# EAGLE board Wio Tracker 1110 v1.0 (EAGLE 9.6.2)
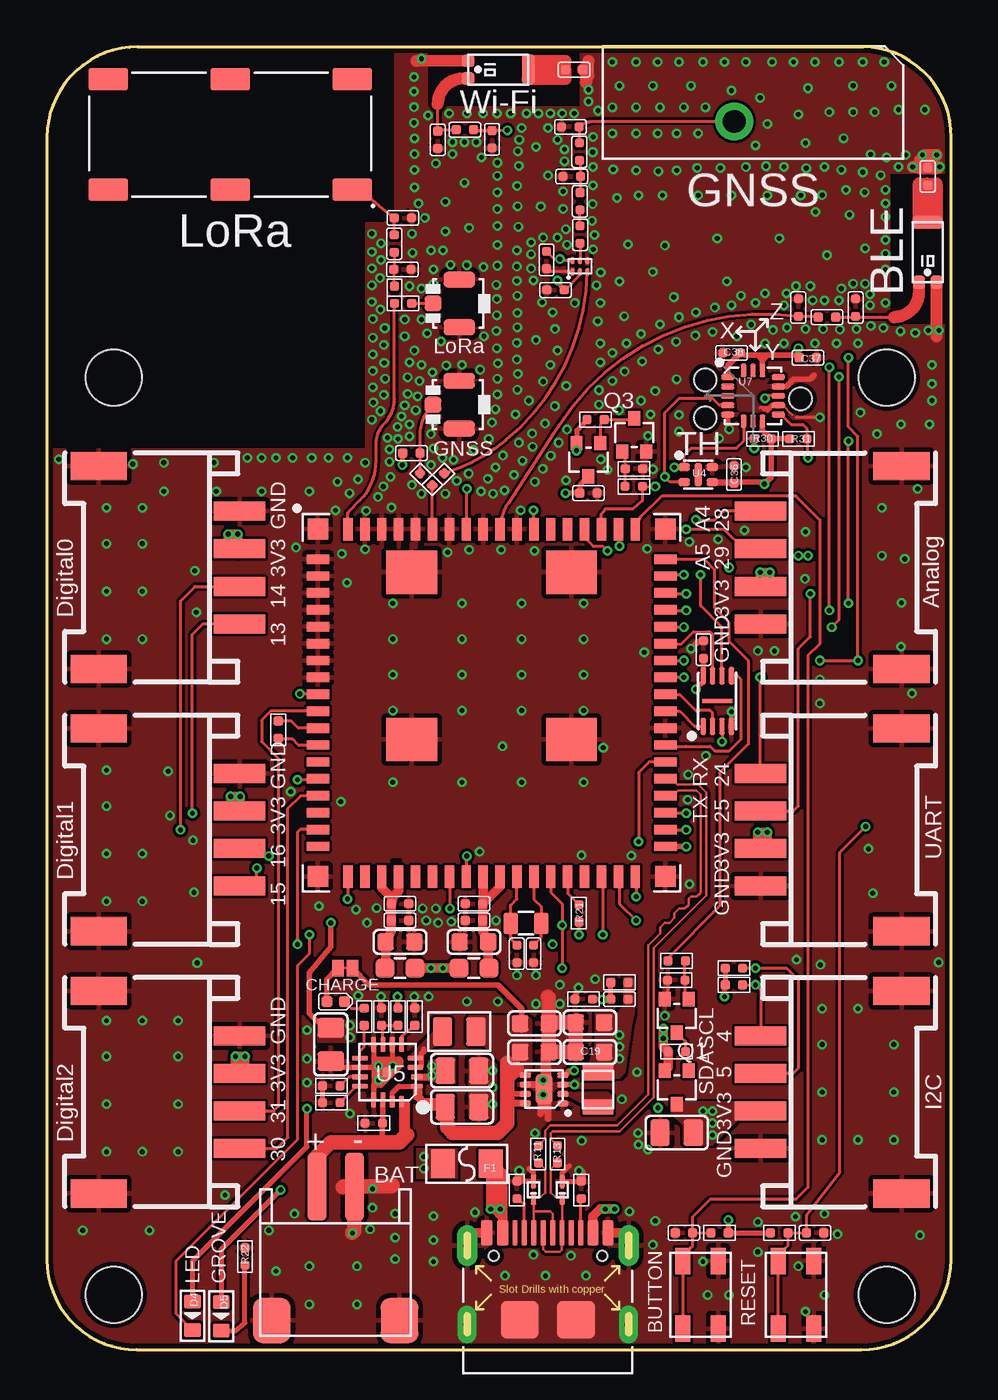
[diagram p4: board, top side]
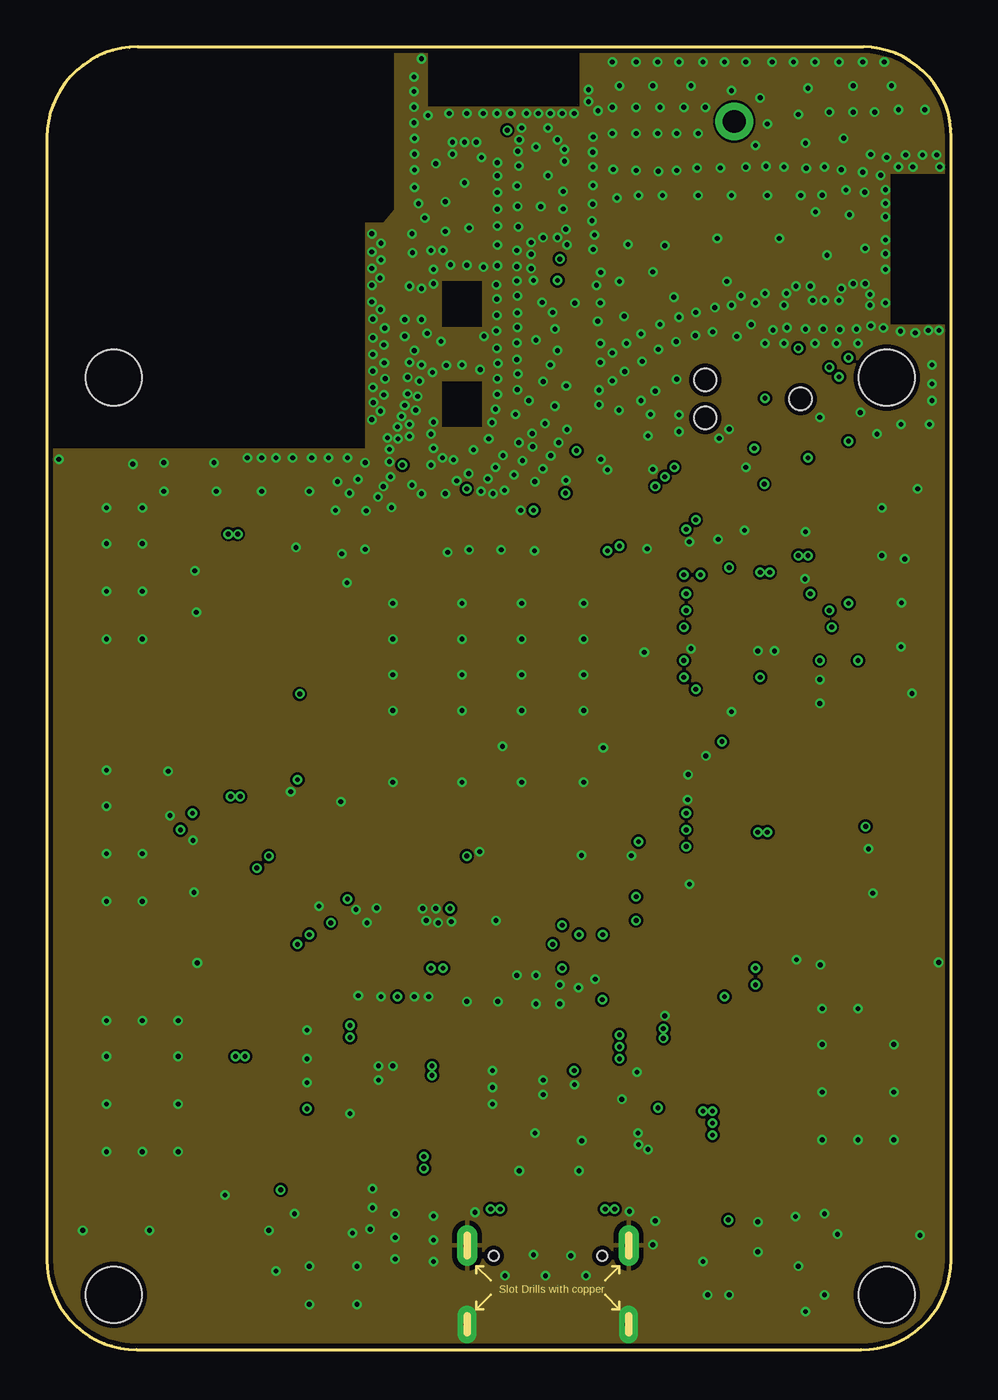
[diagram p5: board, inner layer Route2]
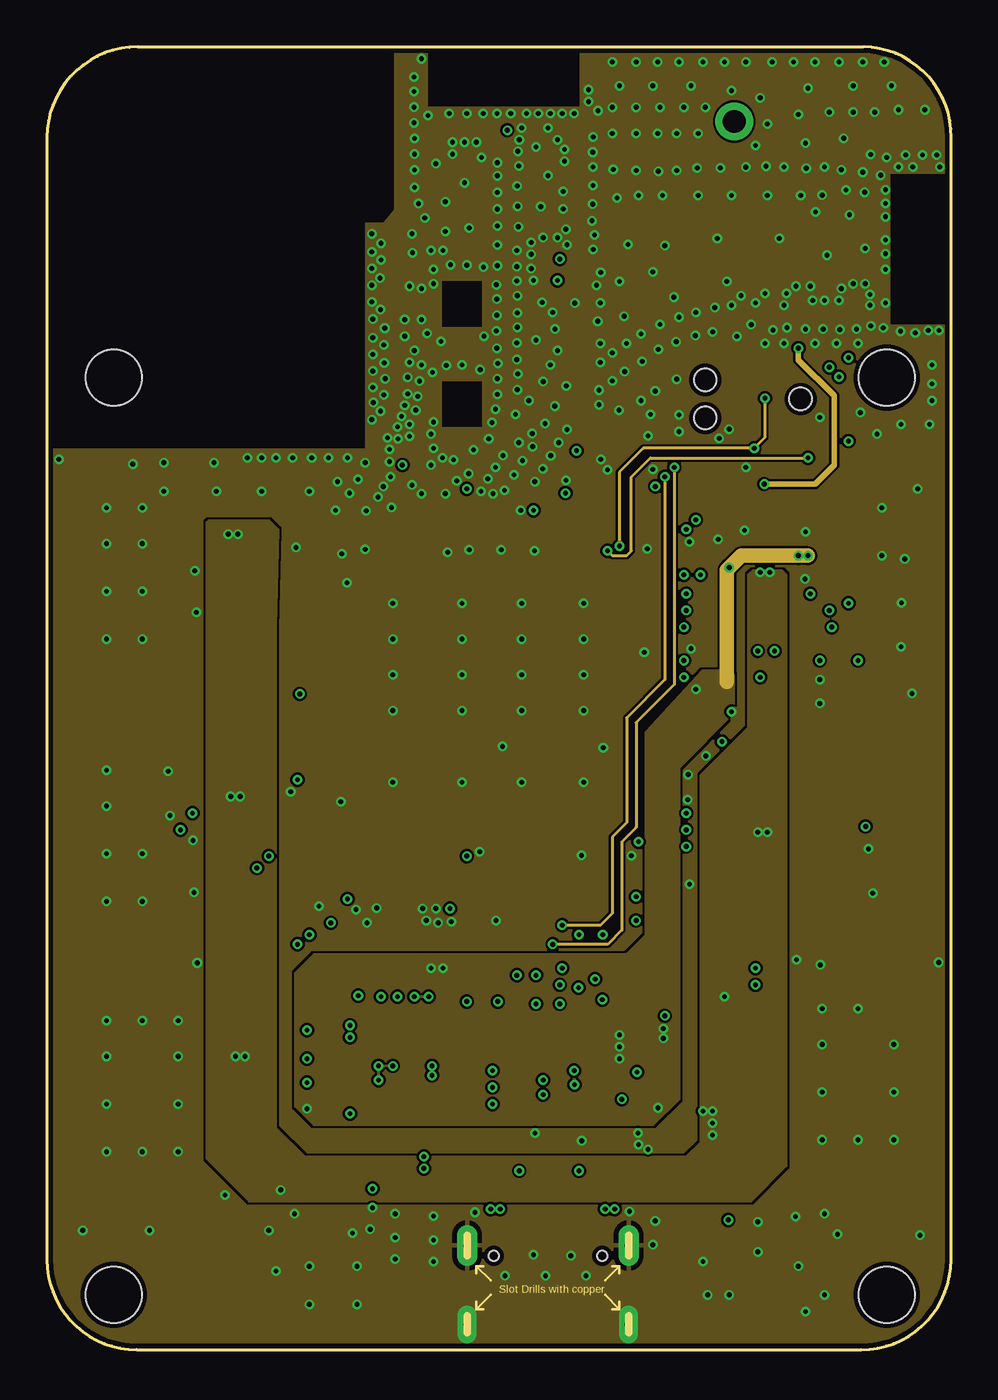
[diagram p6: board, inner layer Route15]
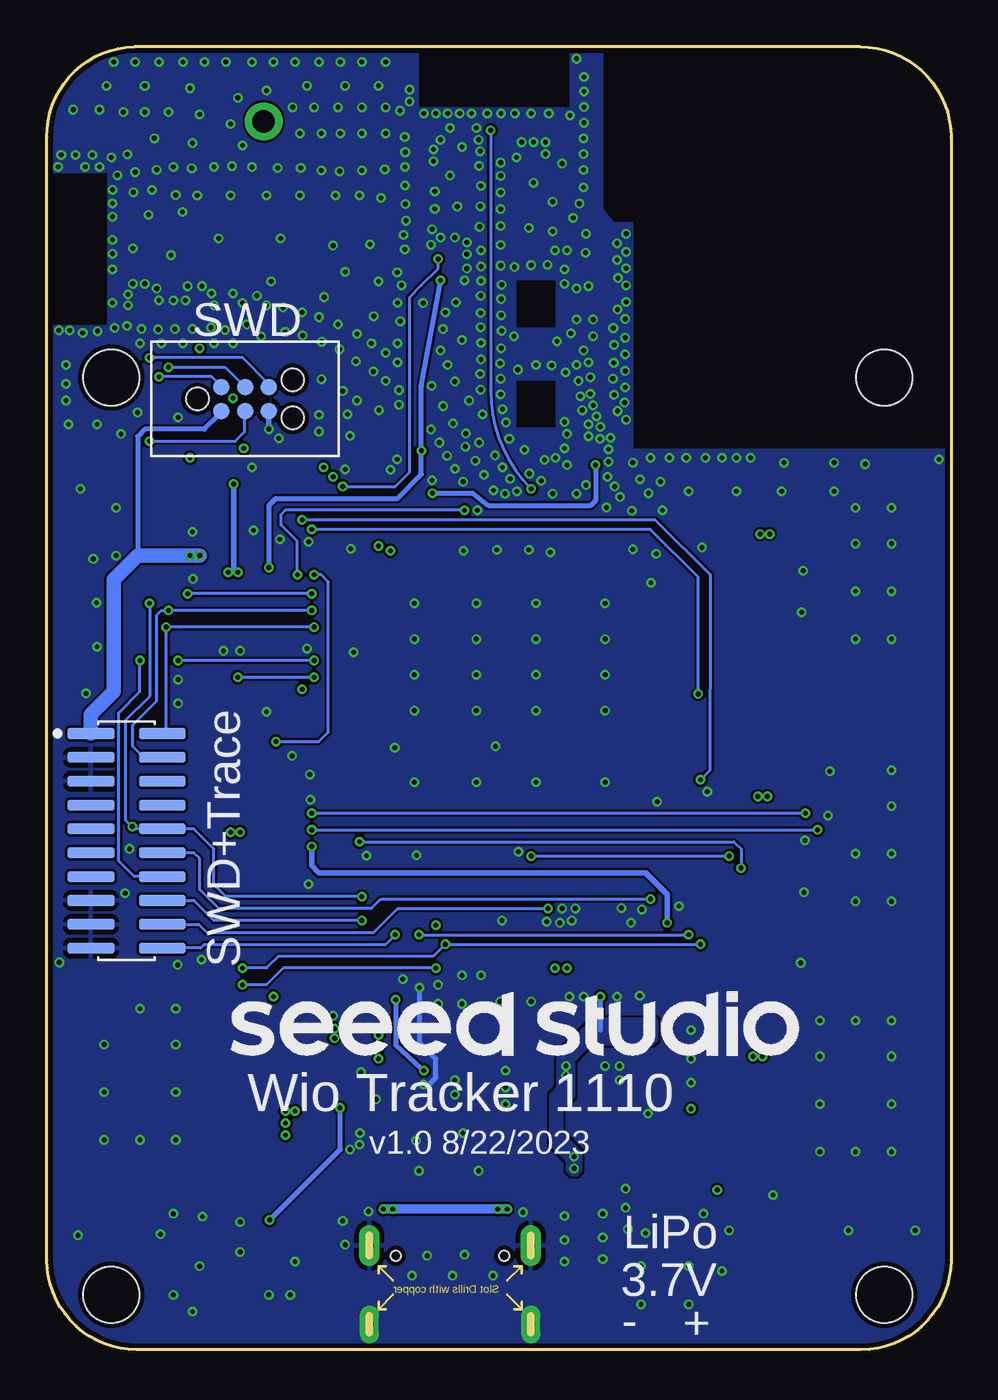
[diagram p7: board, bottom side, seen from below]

Size 48.13 x 69.38 mm. Coordinates in mm from the lower left corner, seen from the top.
Outline: 0,64.58 0,4.78 arc90 4.78,0 43.35,0 arc90 48.13,4.78 48.13,64.58 arc90 43.48,69.38 4.83,69.38 arc90 0,64.58
Copper layers (1*2*15*16): Top 0.035mm / dielectric 0.2mm / Route2 0.0175mm / dielectric 0.3mm / Route15 0.0175mm / dielectric 0.2mm / Bottom 0.035mm
Design rules "SeeedStudio_4layer_DRU_no_angle_20140221 *": minimum track width 1mil, minimum drill 10mil, track to track 5mil, track to pad 5mil, pad to pad 5mil, via to via 5mil, smd to smd 0mil, copper to edge 10mil, drill to drill 8mil, minimum pad ring 4mil, minimum via ring 4mil, stop-mask expansion 4mil, vias tented up to drill 25mil, thermal gap 10mil
Holes 3 mm at 3.56,2.92 44.7,2.92 3.56,51.77 44.7,51.77
tRestrict: area 18.4,24.5 to 18.8,26

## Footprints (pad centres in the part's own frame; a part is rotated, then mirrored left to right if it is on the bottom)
U-FL3P-SMD-2.6X2.6X1.0MM = smd 0.889 x 0.838: D -1.397,0 | smd 1.676 x 0.838: GND1 0,1.27; GND2 0,-1.27
ANT-SMD3P-3.1X1.6X1.04MM = smd 0.65 x 0.7: 1 -0.47,1.6; 2 0.47,1.6 | smd 1.6 x 0.7: 3 0,-1.6
ANT-DIP-14X6X4MM = drill 1.2 pad 2: 1 -1,-1
ANT6-SMD-15X6.5X1.63MM = smd 2.1 x 1.2: 1 -6.5,2.95; 2 0,2.95; 3 6.5,2.95; 4 6.5,-2.95; 5 0,-2.95; 6 -6.5,-2.95
C0402 = smd 0.5 x 0.5: 1 -0.463,0; 2 0.463,0
C0603 = smd 0.889 x 0.889: 1 -0.762,0; 2 0.762,0
C0805 = smd 1.016 x 1.397: 1 -0.889,0; 2 0.889,0
R0402 = smd 0.5 x 0.5: 1 -0.463,0; 2 0.463,0
H2X10-1.27-12.7X3X5.7MM = smd 0.6 x 2.5: 1 -5.715,-1.9; 2 -5.715,1.9; 3 -4.445,-1.9; 4 -4.445,1.9; 5 -3.175,-1.9; 6 -3.175,1.9; 7 -1.905,-1.9; 8 -1.905,1.9; 9 -0.635,-1.9; 10 -0.635,1.9; 11 0.635,-1.9; 12 0.635,1.9; 13 1.905,-1.9; 14 1.905,1.9; 15 3.175,-1.9; 16 3.175,1.9; 17 4.445,-1.9; 18 4.445,1.9; 19 5.715,-1.9; 20 5.715,1.9
SOD-923 = smd 0.7 x 0.3: 1 -0.45,0; 2 0.45,0
LED-0402 = smd 0.58 x 0.58: + -0.468,0; - 0.468,0
LED-0603 = smd 0.762 x 0.889: + -0.762,0; - 0.762,0
FS1206 = smd 1.27 x 1.524: 1 -1.27,0; 2 1.27,0
F0603 = smd 1 x 1: 1 -0.8,0; 2 0.8,0
CONNECTER6P-1.27-9.9X6.1MM = smd 0.88 x 0.88: 1 -1.27,-0.635; 2 -1.27,0.635; 3 0,-0.635; 4 0,0.635; 5 1.27,-0.635; 6 1.27,0.635 | hole 1.2: -2.54,0; 2.54,1.016; 2.54,-1.016
HW2-SMD-2.0-90D = smd 2 x 2.4: 3 3.4,-2.181; 4 -3.4,-2.181 | smd 1 x 3.6: + -1,4.953; - 1,4.953
HW4-SMD-2.0-90D = smd 1.01 x 2.74: 1 -3,-0.1; 2 -1,-0.1; 3 1,-0.1; 4 3,-0.1 | smd 1.5 x 3: SS1 -5.4,7.4; SS2 5.4,7.4
2P-SMD-SHORT = smd 0.61 x 0.889: 1 -0.381,0; 2 0.381,0
SW4P-SMD-4.5X3.2X2.5MM = smd 1.4 x 0.8: 1 -1.8,-0.94; 2 1.8,-0.94; 3 1.8,0.94; 4 -1.8,0.94
L0402 = smd 0.5 x 0.5: 1 -0.463,0; 2 0.463,0
L0806 = smd 1.016 x 1.524: 1 -0.889,0; 2 0.889,0
L201610@1 = smd 0.8 x 1.6: 1 -0.9,0; 2 0.9,0
SOT-323 = smd 0.762 x 0.635: 1 0.889,-0.635; 2 0.889,0.635; 3 -0.889,0
MODULE72_0D9_20X20X2MM = smd 1.2 x 0.5: 1 -9.25,7.65; 2 -9.25,6.75; 3 -9.25,5.85; 4 -9.25,4.95; 5 -9.25,4.05; 6 -9.25,3.15; 7 -9.25,2.25; 8 -9.25,1.35; 9 -9.25,0.45; 10 -9.25,-0.45; 11 -9.25,-1.35; 12 -9.25,-2.25; 13 -9.25,-3.15; 14 -9.25,-4.05; 15 -9.25,-4.95; 16 -9.25,-5.85; 17 -9.25,-6.75; 18 -9.25,-7.65; 37 9.25,-7.65; 38 9.25,-6.75; 39 9.25,-5.85; 40 9.25,-4.95; 41 9.25,-4.05; 42 9.25,-3.15; 43 9.25,-2.25; 44 9.25,-1.35; 45 9.25,-0.45; 46 9.25,0.45; 47 9.25,1.35; 48 9.25,2.25; 49 9.25,3.15; 50 9.25,4.05; 51 9.25,4.95; 52 9.25,5.85; 53 9.25,6.75; 54 9.25,7.65 | smd 0.5 x 1.2: 19 -7.65,-9.25; 20 -6.75,-9.25; 21 -5.85,-9.25; 22 -4.95,-9.25; 23 -4.05,-9.25; 24 -3.15,-9.25; 25 -2.25,-9.25; 26 -1.35,-9.25; 27 -0.45,-9.25; 28 0.45,-9.25; 29 1.35,-9.25; 30 2.25,-9.25; 31 3.15,-9.25; 32 4.05,-9.25; 33 4.95,-9.25; 34 5.85,-9.25; 35 6.75,-9.25; 36 7.65,-9.25; 55 7.65,9.25; 56 6.75,9.25; 57 5.85,9.25; 58 4.95,9.25; 59 4.05,9.25; 60 3.15,9.25; 61 2.25,9.25; 62 1.35,9.25; 63 0.45,9.25; 64 -0.45,9.25; 65 -1.35,9.25; 66 -2.25,9.25; 67 -3.15,9.25; 68 -4.05,9.25; 69 -4.95,9.25; 70 -5.85,9.25; 71 -6.75,9.25; 72 -7.65,9.25 | smd 1.1 x 1.1: 73 -9.25,9.25; 74 -9.25,-9.25; 75 9.25,-9.25; 76 9.25,9.25 | smd 2.7 x 2.3: 77 -4.25,6.95; 78 -4.25,-1.95; 79 4.25,-1.95; 80 4.25,6.95
USON8-0.5-3X2MM = smd 0.9 x 0.3: 1 -1.35,0.75; 2 -1.35,0.25; 3 -1.35,-0.25; 4 -1.35,-0.75; 5 1.35,-0.75; 6 1.35,-0.25; 7 1.35,0.25; 8 1.35,0.75 | smd 0.2 x 1.6: BP 0,0
BGA6-0.4-1.1X0.7X0.4MM = smd 0.4 x 0.2: 1 -0.3,0.4; 2 -0.3,0; 3 -0.3,-0.4; 4 0.3,-0.4; 5 0.3,0; 6 0.3,0.4
SNR4-0.8-1.5X1.5X0.54MM = smd 0.6 x 0.4: 1 -0.75,0.4; 2 -0.75,-0.4; 3 0.75,-0.4; 4 0.75,0.4 | smd 0.4 x 1.2: 5 0,0
QFN16G-0.5-3X3MM = smd 0.65 x 0.28: 1 -1.575,0.75; 2 -1.575,0.25 | smd 0.85 x 0.28: 3 -1.475,-0.25; 4 -1.475,-0.75; 9 1.475,-0.75; 10 1.475,-0.25; 11 1.475,0.25; 12 1.475,0.75 | smd 0.28 x 0.85: 5 -0.75,-1.475; 6 -0.25,-1.475; 7 0.25,-1.475; 8 0.75,-1.475; 13 0.75,1.475; 14 0.25,1.475 | smd 0.28 x 0.65: 15 -0.25,1.575; 16 -0.75,1.575 | smd 0.508 x 0.508: PAD 0,0
DFN8G-0.5-2X2MM = smd 0.6 x 0.3: 1 -1,0.75; 2 -1,0.25; 3 -1,-0.25; 4 -1,-0.75; 5 1,-0.75; 6 1,-0.25; 7 1,0.25; 8 1,0.75 | smd 0.9 x 1.6: 9 0,0
LGA16-0.5-3X3MM = smd 0.7 x 0.3: 1 -1.35,0.873; 2 -1.35,0.373; 3 -1.35,-0.127; 4 -1.35,-0.627; 5 -1.35,-1.127; 9 1.35,-1.127; 10 1.35,-0.627; 11 1.35,-0.127; 12 1.35,0.373; 13 1.35,0.873 | smd 0.3 x 0.7: 6 -0.5,-1.477; 7 0,-1.477; 8 0.5,-1.477; 14 0.5,1.223; 15 0,1.223; 16 -0.5,1.223
USB2.0-TYPE-C = smd 1.35 x 0.6: A1_B12 0.125,3.25; A4_B9 0.125,2.4; B1_A12 0.125,-3.2; B4_A9 0.125,-2.4 | smd 1.35 x 0.3: A5 0.125,1.25; A6 0.125,0.25; A7 0.125,-0.25; A8 0.125,-1.25; B5 0.125,-1.75; B6 0.125,-0.75; B7 0.125,0.75; B8 0.125,1.75 | drill 0.4 pad 1 long: S1 -4.75,4.3; S2 -4.75,-4.3 | drill 0.4 pad 1.1 long: S3 -0.55,4.3; S4 -0.55,-4.3 | smd 2 x 2: S5 -4.5,1.5; S6 -4.5,-1.5 | hole 0.55: -1.1,-2.89; -1.1,2.89
X2-SMD-L2.0X1.2X0.55MM = smd 0.762 x 1.143: 1 -0.813,0; 2 0.813,0

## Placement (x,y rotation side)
ANT1  U.FL-R-SMT-1  [U-FL3P-SMD-2.6X2.6X1.0MM]  21.95,55.72 0 top
ANT2  U.FL-R-SMT-1  [U-FL3P-SMD-2.6X2.6X1.0MM]  21.94,50.33 0 top
ANT3  RFECA3216060A1T  [ANT-SMD3P-3.1X1.6X1.04MM]  24.03,68.17 90 top
ANT4  RFECA3216060A1T  [ANT-SMD3P-3.1X1.6X1.04MM]  46.89,58.45 180 top
ANT5  M04-0103010R0A  [ANT-DIP-14X6X4MM]  37.59,66.42 0 top
ANT6  MD1506  [ANT6-SMD-15X6.5X1.63MM]  9.75,64.72 180 top
C1  7.5pF  [C0402]  18.92,57.53 180 top
C2  DNP  [C0402]  18.95,60.27 180 top
C3  1.2pF  [C0402]  27.94,62.48 0 top
C4  DNP  [C0402]  27.86,65.12 0 top
C5  1.2pF  [C0402]  23.7,64.46 90 top
C6  0.5pF  [C0402]  20.8,64.44 90 top
C7  1.2pF  [C0402]  40.01,55.5 270 top
C8  0.5pF  [C0402]  43.05,55.5 270 top
C9  1nF  [C0402]  28.07,68.17 180 top
C10  1nF  [C0402]  46.89,62.48 270 top
C11  47pF  [C0402]  22.73,23.75 0 top
C12  100nF  [C0402]  22.73,22.86 0 top
C13  10uF  [C0603]  22.73,21.72 0 top
C14  47pF  [C0402]  18.8,22.86 180 top
C15  100nF  [C0402]  18.8,23.75 180 top
C16  10uF  [C0603]  18.8,21.72 180 top
C17  12pF  [C0402]  25.02,21.08 90 top
C18  10uF  [C0805]  33.53,11.56 180 top
C19  10uF  [C0603]  28.91,15.85 0 top
C20  12pF  [C0402]  25.91,21.08 90 top
C21  10uF  [C0603]  25.96,17.37 180 top
C22  10uF  [C0805]  22.1,14.86 0 top
C23  10uF  [C0805]  15.11,16.26 270 top
C24  10uF  [C0805]  22.1,12.93 0 top
C25  1uF  [R0402]  17.4,12.06 180 top
C26  10uF  [C0603]  28.91,17.42 0 top
C27  10uF  [C0603]  25.96,15.85 180 top
C28  100nF  [C0402]  33.91,6.22 0 top
C29  100nF  [C0402]  40.89,6.22 180 top
C30  100nF  [C0402]  34.95,37.29 270 top
C31  1nF  [C0402]  27.08,56.44 0 top
C32  1nF  [C0402]  26.59,58.04 90 top
C33  100nF  [C0402]  28.83,45.62 180 top
C34  1nF  [C0402]  28.37,61.16 270 top
C35  1nF  [C0402]  30.48,18.67 0 top
C36  100nF  [C0402]  36.58,46.61 270 top
C37  100nF  [C0402]  40.51,52.83 180 top
C38  100nF  [C0402]  36.45,53.09 0 top
CN1  DNP  [H2X10-1.27-12.7X3X5.7MM]  43.89,27.1 270 bottom
D1  DF2S6.8FS  [SOD-923]  27.43,8.51 90 top
D2  DF2S6.8FS  [SOD-923]  25.91,8.51 90 top
D3  Green  [LED-0402]  15.37,18.54 0 top
D4  Blue  [LED-0603]  7.75,1.8 270 top
D5  Red  [LED-0603]  9.27,1.78 270 top
F1  750mA  [FS1206]  22.35,9.91 180 top
FB1  BLM18PG121SN1D  [F0603]  22.73,20.32 180 top
FB2  BLM18PG121SN1D  [F0603]  18.8,20.32 0 top
FR1  SEEEDSTUDIO-OPEN-SCH-FRAME  [SEEEDSTUDIO-PCB-FRAME]  not placed on the board
FR2  SEEEDSTUDIO-OPEN-SCH-FRAME  [SEEEDSTUDIO-PCB-FRAME]  not placed on the board
FR3  SEEEDSTUDIO-OPEN-SCH-FRAME  [SEEEDSTUDIO-PCB-FRAME]  not placed on the board
FR4  SEEEDSTUDIO-OPEN-SCH-FRAME  [SEEEDSTUDIO-PCB-FRAME]  not placed on the board
J1  [CONNECTER6P-1.27-9.9X6.1MM]  37.59,50.63 0 bottom
J2  JST-2P-SMD-90D  [HW2-SMD-2.0-90D]  15.37,3.73 0 top
J3  SMD Grove  [HW4-SMD-2.0-90D]  38.1,27.69 270 top
J4  SMD Grove  [HW4-SMD-2.0-90D]  10.16,41.66 90 top
J5  SMD Grove  [HW4-SMD-2.0-90D]  10.16,13.72 90 top
J6  SMD Grove  [HW4-SMD-2.0-90D]  38.1,41.66 270 top
J7  SMD Grove  [HW4-SMD-2.0-90D]  10.16,27.69 90 top
J8  SMD Grove  [HW4-SMD-2.0-90D]  38.1,13.72 270 top
JP1  [2P-SMD-SHORT]  15.88,20.32 0 top
K1  SKRPABE010  [SW4P-SMD-4.5X3.2X2.5MM]  34.8,2.92 90 top
K2  SKRPABE010  [SW4P-SMD-4.5X3.2X2.5MM]  39.88,2.92 90 top
L1  18nH  [L0402]  18.49,58.9 90 top
L2  1.2pF  [L0402]  28.35,63.8 90 top
L3  2.2uH  [L0806]  21.95,16.94 0 top
L4  0.47uH  [L201610@1]  29.34,13.84 90 top
L5  5.6nH  [L0402]  22.25,64.97 180 top
L6  4.7nH  [L0402]  41.53,54.99 0 top
L7  27nH  [L0402]  19.41,47.75 0 top
L8  8.2nH  [L0402]  28.38,59.38 90 top
Q1  2N7002PW  [SOT-323]  33.53,17.78 90 top
Q2  CJ2101  [SOT-323]  33.53,13.97 90 top
Q3  2N7002PW  [SOT-323]  31.27,48.72 270 top
Q4  CJ2101  [SOT-323]  28.83,47.4 90 top
R1  5.1K  [R0402]  25.02,8.51 270 top
R2  5.1K  [R0402]  28.45,8.51 270 top
R3  0R  [R0402]  18.5,56.18 90 top
R4  DNP  [R0402]  18.96,55.73 0 top
R5  0R  [R0402]  20.83,46.35 45 top
R6  DNP  [R0402]  20.19,46.35 135 top
R7  0R  [R0402]  12.32,33.02 90 top
R8  10k  [R0402]  38.99,6.22 180 top
R9  10k  [R0402]  35.81,6.22 0 top
R10  1k  [R0402]  31.24,45.97 0 top
R11  22R  [R0402]  26.16,10.41 90 top
R12  100k  [R0402]  29.21,49.53 180 top
R13  22R  [R0402]  27.18,10.41 90 top
R14  10k  [R0402]  36.58,19.43 180 top
R15  0R  [R0402]  19.58,17.73 90 top
R16  DNP  [R0402]  18.69,17.73 270 top
R17  2K  [R0402]  16.89,17.73 270 top
R18  0R  [R0402]  17.81,17.73 90 top
R19  2K  [R0402]  15.14,13.16 180 top
R20  2K  [R0402]  15.14,14.05 180 top
R21  1k  [R0402]  28.32,23.24 90 top
R22  1k  [R0402]  10.54,4.97 90 top
R23  1k  [R0402]  33.53,20.7 180 top
R24  100k  [R0402]  33.53,15.88 180 top
R25  10k  [R0402]  36.58,20.32 180 top
R26  100k  [R0402]  33.5,19.69 0 top
R27  100k  [R0402]  31.25,46.91 180 top
R28  100K  [R0402]  30.48,19.56 0 top
R29  22K  [R0402]  28.57,18.67 0 top
R30  DNP  [R0402]  38.1,48.51 0 top
R31  DNP  [R0402]  40.01,48.51 180 top
U1  WM1110-A  [MODULE72_0D9_20X20X2MM]  23.67,34.45 0 top
U2  P25Q32SH-UXH-IR  [USON8-0.5-3X2MM]  35.69,34.54 90 top
U3  BGA524N6  [BGA6-0.4-1.1X0.7X0.4MM]  28.37,57.71 90 top
U4  SHT41  [SNR4-0.8-1.5X1.5X0.54MM]  34.67,46.61 0 top
U5  ETA6003  [QFN16G-0.5-3X3MM]  18.14,14.78 180 top
U6  ETA3410  [DFN8G-0.5-2X2MM]  26.47,13.87 180 top
U7  LIS3DHTR  [LGA16-0.5-3X3MM]  37.59,50.93 0 top
U$8  [LOGO-SEEED-NEW-3X30MM]  38.35,15.62 0 bottom
USB1  UBF31-0171  [USB2.0-TYPE-C]  26.67,6.1 90 top
X1  32.768KHz  [X2-SMD-L2.0X1.2X0.55MM]  25.5,22.71 180 top

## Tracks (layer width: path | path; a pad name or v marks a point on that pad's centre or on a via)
3V3  (via drill 0.25 pad 0.51)
  Top 0.152: 34.94,36.94 C30.2
  Top 0.156: U3.2 28.37,57.23 27.56,56.42
  Top 0.254: 34.94,36.94 U2.8 34.94,35.57 v34.54,35.18 | v13.84,12.83 13.84,10.79 7.75,4.7 D4.+ | v36.28,6.91 R9.2 R8.2 | C31.2 27.56,56.42 v27.18,56.94 | R12.2 28.19,48.95 Q4.2 v28.19,47.88
  Top 0.508: FB2.2 v20.45,20.32 v21.08,20.32 FB1.2 | Q2.2 33.07,15.03 R24.2 32.82,16.12 v32.82,17.09
  Route15 0.762: v40.51,42.29 v40.01,42.29 36.96,42.29 v36.32,41.66 36.2,41.53 36.2,35.56
  Bottom 0.254: v36.32,41.66 36.32,44.96 35.94,45.34 29.46,45.34 28.19,46.61 v28.19,47.88 28.19,51.31 v27.18,56.94 | v36.28,6.91 v36.27,6.91 32.51,10.67 32.51,12.98 v32.54,12.88 | J1.1 38.86,49.79 38.86,49.78 38.99,49.78 39.75,49.02 42.93,49.02 43.31,48.64 43.31,42.29
  Bottom 0.762: CN1.1 45.79,33.84 44.58,35.05 44.58,41.02 43.31,42.29 v40.51,42.29 v40.01,42.29
  other vias: 30.48,16.76 30.48,16.13 30.48,15.49 32.82,16.59
  pour Top (no thermals): 28.7,14.61 29.21,16.26 29.21,17.91 30.35,17.91 30.73,18.29 30.73,19.81 31.24,19.81 31.24,17.91 31.11,17.4 30.73,14.73 30.48,14.48 28.83,14.48
  pour Route15: 34.92,36.2 36.32,36.2 36.58,35.94 36.58,33.91 33.66,30.99 33.66,13.34 32.26,11.94 14.22,11.94 13.21,12.95 13.21,20.07 14.22,21.08 30.86,21.08 31.88,22.1 31.88,32.89
3V3B  (via drill 0.25 pad 0.51)
  Top 0.254: R25.2 R14.2 | R14.2 36.2,19.43 | v12.45,8.51 9.27,5.33 D5.+ | R14.2 36.07,19.38 v36.07,18.8
  Top 0.305: U7.8 38.09,48.98 R30.2 | R31.2 R30.2 | R30.2 38.56,46.47 v38.19,46.1 | 37.85,52.96 37.97,52.96 | 37.97,52.96 38.35,52.96 | 38.35,52.96 39.92,52.96 C37.2 40.01,52.88 v40.01,53.34 | 38.15,46.15 v38.19,46.1 | U7.14 38.09,52.7 | 38.09,52.71 38.09,52.84 37.97,52.96 | 38.09,52.7 38.09,52.71 | 38.09,52.71 37.85,52.96 | 38.09,52.7 38.35,52.96 | v38.19,46.1 38.19,46.21 U4.3 35.42,46.15 C36.2 | 37.85,52.96 37.17,52.96 C38.2 36.24,52.42 U7.1
  Top 0.508: 38.48,40.51 v38.48,41.4 v37.97,41.4 37.97,40.68 J6.3 | J3.3 37.85,26.97 v37.85,27.56 v38.35,27.56 38.35,26.91 J3.3 | J5.3 10.54,15 v10.54,15.62 v10.03,15.62 10.03,14.94 J5.3 | J7.3 9.78,28.56 v9.78,29.46 v10.29,29.46 10.29,28.61 J7.3 | J4.3 9.65,42.5 v9.65,43.43 v10.16,43.43 10.16,42.4 J4.3
  Route15 0.305: v40.01,53.34 40.01,52.7 41.91,50.8 41.91,47.12 40.89,46.1 v38.19,46.1 38.15,46.15
  Bottom 0.305: v38.19,46.1 38.19,41.62 v37.97,41.4
  other vias: 35.43,12.7 35.43,12.06 35.43,11.43 34.92,12.7
  pour Top (no thermals): 33.4,13.21 38.23,13.21 38.35,13.08 38.35,12.45 38.23,12.32 36.83,12.32 35.43,10.92 34.04,10.92 33.91,11.05 33.91,11.94 33.27,12.57 33.27,13.08
  pour Route15: 8.64,44.2 11.81,44.2 12.32,43.69 12.19,38.48 12.19,11.81 13.72,10.29 34.04,10.29 34.8,11.05 34.8,30.61 37.34,33.15 37.34,41.27 37.59,41.53 39.12,41.53 39.37,41.27 39.37,9.78 37.47,7.87 10.79,7.87 8.51,10.16 8.51,44.07
GND  (via drill 0.25 pad 0.51)
  Top 0.102: 39.17,50.3 39.69,49.78
  Top 0.127: U7.10 39.17,50.3
  Top 0.152: U3.1 26.76,57.41 C32.1 | 39.88,49.66 v41.15,49.66 | 38.35,50.16 37.97,50.16
  Top 0.156: R26.1 33.02,18.6 | 26.66,57.51 C32.1
  Top 0.254: R29.1 28.29,19.2 v28.29,19.28 | R18.2 17.78,18.11 v17.78,18.8 | R15.2 19.56,18.11 v19.56,18.8 | U2.4 v36.45,33.97 | U5.10 17.89,15.03 U5.PAD | R19.2 R20.2 | U5.8 17.39,15.51 17.78,15.11 17.91,15.11 v17.65,14.35 18.39,15.08 U5.6 | R2.1 28.38,8.96 D1.2 27.43,9.4 27.81,9.78 | 25.15,9.02 25.2,8.96 D2.2 25.91,9.4 25.65,9.65 | 38.35,50.1 38.16,50.1 | U7.10 38.62,50.3 38.35,50.04
  Top 0.305: U6.3 v28.09,14.12 | C23.2 15.55,15.03 U5.10 17.99,15.03 v17.65,14.35 17.39,14.08 U5.13 | C30.1 34.67,37.72 v34.29,37.34 | U7.12 39.36,51.3 39.75,51.69 40.64,51.69 40.85,51.9 | U7.5 36.24,49.1 v36.32,49.02
  Top 0.381: U6.6 26.22,14.12 U6.9 | U6.9 26.47,14.78 | 26.47,14.78 26.67,14.99 | 26.67,14.99 26.67,15.62 | 26.67,14.99 26.67,14.35 | 26.47,14.78 26.47,15.67 26.54,15.75 | U6.9 26.29,13.69 26.29,12.57 | U6.9 26.67,13.66 26.67,12.32
  Top 0.508: USB1.A1_B12 22.48,6.22 22.35,6.1 22.35,5.56 USB1.S3 | R1.1 25.15,9.02 v25.15,9.53 | R2.1 28.45,9.4 v28.32,9.53 | USB1.B1_A12 30.61,6.22 30.99,5.84 30.99,5.56 USB1.S4
  Top 0.635: ANT3.2 19.68,68.63 | C9.1 28.7,68 28.7,67.74 | 28.7,67.74 28.7,67.48 | 28.7,67.74 28.83,67.87 28.83,68.63 | ANT4.1 47.36,53.98 47.37,53.98 | v46.1,62.99 46.35,62.99 | 46.35,62.99 47.47,62.99 | v47.37,63.63 46.74,63.63 46.48,63.37 | 46.35,62.99 46.42,62.93 47.43,62.93
  Top 0.762: J2.- 18.34,8.69 18.41,8.76 | J2.- 16.37,6.33 16.26,6.22 | J2.- 15.8,8.69 15.75,8.64 | C27.1 26.72,17.22 | 26.72,17.22 26.67,17.27 | 26.72,17.22 26.72,18.74 26.67,18.8 | C26.1 26.82,17.42 26.8,17.4 | 26.67,16 26.82,15.85 C19.1 28.14,17.48 28.19,17.53
  Bottom 0.254: v28.09,14.12 27.79,14.12 27.43,14.48 27.43,15.49 28.29,16.36 v28.29,19.28
  Bottom 0.305: v36.32,49.02 J1.5
  other vias: 23.72,14.86 23.72,13.97 23.72,13.08 36.32,2.92 13.84,15.49 13.84,14.22 16.13,12.57 13.84,17.02 20.32,18.8 22.35,18.54 24,18.54 14.48,23.62 20.83,22.73 20.19,22.86 20.7,23.49 17.55,23.52 17.04,22.73 26.04,19.94 27.3,19.43 31.42,14.78 26.04,18.41 27.3,18.41 30.61,13.34 29.18,19.74 3.17,17.53 3.17,13.08 3.17,10.54 3.17,15.62 5.08,17.53 25.91,5.05 25.98,11.53 5.08,10.54 6.99,10.54 6.99,13.08 6.99,15.62 6.99,17.53 3.17,44.83 3.17,40.39 3.17,37.85 3.17,42.93 5.08,44.83 5.08,42.93 5.08,40.39 5.08,37.85 3.17,30.86 3.17,26.42 3.17,23.88 3.17,28.96 6.45,30.81 6.55,28.45 5.08,26.42 5.08,23.88 41.27,18.16 41.27,13.72 41.27,11.18 41.27,16.26 43.18,18.16 34.21,24.79 27.89,5 43.18,11.18 44.45,44.83 46.35,45.85 45.67,42.11 45.49,39.78 45.47,37.44 44.45,42.29 45.47,49.28 46.99,49.28 18.41,39.75 18.41,37.85 18.41,35.94 18.41,34.04 22.1,39.75 22.1,37.85 22.1,35.94 22.1,34.04 25.27,39.75 25.27,37.85 25.27,35.94 25.27,34.04 28.57,39.75 28.57,37.85 28.57,35.94 28.57,34.04 18.41,30.23 22.1,30.23 25.27,30.23 28.57,30.23 47.12,52.45 47.12,51.43 47.12,50.55 11.43,47.5 13.97,45.72 11.43,45.72 10.67,47.5 8.89,47.24 9.02,45.72 6.22,45.72 6.22,47.24 37.21,46.99 40.39,43.56 7.82,24.36 9.47,8.23 7.77,27.13 8,20.6 12.19,4.19 13.97,4.45 16.51,4.45 16.51,2.41 13.97,2.41 20.57,7.11 20.57,5.84 20.57,4.7 18.54,7.24 18.54,5.97 18.54,4.83 32.38,6.86 32.26,5.59 46.48,6.1 42.09,6.15 37.85,5.21 28.47,11.13 31.47,11.53 43.56,58.65 46.23,54.15 41.27,61.49 42.55,61.77 44.64,61.04 44.64,61.78 41.4,62.99 42.29,62.84 43.43,62.71 43.54,61.65 32.89,17.78 21.42,65.83 22.35,65.83 20.29,65.73 23.22,65.83 23.96,65.83 24.69,65.83 37.85,37.21 38.73,37.21 19.94,68.76 19.54,67.78 19.54,67.01 19.54,66.18 19.54,65.34 19.57,64.51 19.57,63.67 19.57,62.84 19.57,61.9 20.45,58.55 21.08,58.55 21.59,63.67 21.59,64.31 22.23,64.31 22.86,64.31 22.78,7.32 23.14,63.5 23.98,63.22 23.93,56.72 23.98,57.73 23.95,53.34 23.95,55.96 35.79,48.54 23.95,55.09 23.93,54.25 24,52.53 23.98,51.71 23.98,50.88 23.88,50.09 23.7,49.38 23.52,48.51 22.48,42.6 22.71,47.93 7.87,41.48 21.64,47.4 21.06,47.5 20.45,47.12 20.57,49.4 20.45,48.77 20.57,48.01 19.63,50.04 19.3,49.28 19.3,48.64 18.24,47.96 43.97,24.31 19.05,50.29 17.93,53.52 18.01,51.71 13.18,7.24 17.96,52.55 15.98,40.84 16.99,44.68 18.34,44.86 19.94,45.59 18.29,46.48 19.43,46.05 17.63,45.42 21.34,42.47 18.24,47.29 32.26,57.4 19.3,56.64 19.94,56.52 21.21,59.56 20.57,56.77 20.57,57.53 21.49,57.78 17.3,59.44 22.35,57.76 23.24,57.66 23.04,26.52 19.94,54.86 17.78,58.04 19.05,54.86 17.35,54.89 17.75,55.4 17.35,53.9 47.47,20.62 17.73,57.07 46.05,34.95 17.37,50.44 17.3,49.53 41.17,20.5 17.75,49.99 17.93,50.85 16.56,46.35 12.98,29.72 15.47,46.23 16.1,45.62 16.94,42.62 15.37,44.7 19.2,51.79 18.69,48.51 19.84,51.59 19.3,52.58 19.56,53.21 19.05,53.98 17.35,51.26 19.74,50.77 17.3,55.8 20.52,52.04 21.26,52.43 35.08,31.62 22.1,52.45 34.11,29.29 23.06,52.2 19.94,52.45 23.27,53.98 7.95,39.27 34.14,30.63 20.98,53.7 20.24,54.13 21.21,45.59 21.82,46.28 22.45,46.66 23.11,45.72 23.47,46.38 23.88,46.99 24.28,47.62 25.12,48.31 19.46,58.42 25.04,51.13 25.96,42.55 25.07,51.97 25.02,52.73 25.02,53.62 25.04,54.46 25.04,55.22 27.64,46.3 25.02,56.92 39.9,20.78 25.02,57.68 37.85,6.81 25.02,58.55 25.15,64.44 25.27,65.07 25.53,65.83 26.16,65.83 26.8,65.83 27.43,65.83 28.07,65.83 29.34,65.99 28.83,66.47 28.83,67.1 29.08,64.59 29.06,63.78 29.08,58.59 31.01,7.37 29.48,57.38 43.74,26.67 29.26,56.69 19.79,61.04 23.75,45.59 24.36,45.77 26.67,65.07 25.07,63.83 27.18,64.44 27.56,63.93 27.56,63.29 25.12,63.04 25.1,59.8 15.65,29.18 25.06,60.9 27.49,61.69 27.49,60.75 37.13,43.64 29.62,32.05 25.04,56.13 16.46,23.44 25.78,58.98 25.78,58.34 25.78,57.58 29.32,54.78 30.15,62.85 34.2,43.03 31.37,62.8 32.55,62.76 31.8,37.15 33.53,62.8 34.62,62.94 28.46,26.33 35.85,62.94 31.11,26.31 37.21,62.98 38.28,63.03 40.92,60.59 39.24,62.99 39.24,55.63 38.66,54.31 13.26,42.72 40.39,54.36 41.33,54.36 40.36,41.05 42.21,54.33 39.4,54.43 43.1,54.36 43.87,54.52 44.53,54.42 45.44,54.24 46.93,54.29 47.5,54.29 44.64,57.53 44.64,58.37 44.64,59.1 44.64,60.34 44.39,62.55 39.37,56.26 39.88,56.64 40.64,56.64 40.77,55.88 41.4,55.88 42.16,55.88 42.29,56.52 42.93,56.77 43.56,56.77 43.81,56.2 43.81,55.63 29.49,47.42 29.84,46.86 30.45,50.04 32.13,49.81 30.76,52.1 33.53,51.69 30.48,56.9 29.46,55.75 31.5,61.47 30.35,61.34 32.77,61.47 36.96,56.13 36.2,56.9 38.23,56.26 26.04,64.06 25.03,61.98 26.37,55.78 16.57,18.86 42.73,60.44 40.42,62.92 44.64,55.75 25.22,44.7 17.65,15.11 18.41,15.11 26.42,14.35 26.42,13.59 25.02,19.94 21.53,22.8 20,23.49 16.27,6.21 17.21,6.41 17.34,7.56 17.34,8.57 41.4,7.24 39.85,7.09 40.39,2.03 41.4,2.92 35.18,2.92 34.92,4.7 40.01,4.45 24.38,3.94 26.54,3.94 28.7,3.94 24.26,32.13 11.81,6.35 1.91,6.35 5.46,6.35 31.5,10.92 32,10.67 41.15,35.69 41.15,34.42 35.74,43.15 45.09,16.26 45.09,13.72 45.09,11.18 30.94,58.86 29.07,62.99 29.01,60.12 29.05,61.01 29.07,62.01 29.15,59.37 28.11,55.74 27.62,59.67 27.69,58.85 26.42,59.23 27.18,59.23 24.18,42.6 25.91,56.94 20.12,60.27 17.78,58.93 24.94,49.81 19.43,59.44 25.83,48.79 26.52,49.33 27.04,50.25 27.65,51.33 24.87,46.6 25.32,47.35 25.86,48.09 25.97,46.23 26.4,46.91 26.82,47.61 27.24,48.31 27.69,49.01 29.39,50.33 29.39,51.1 30.1,51.6 31.69,52.64 32.55,53.28 33.5,53.68 31.95,42.66 34.52,54.01 35.45,54.2 15.7,42.39 36.73,53.96 33.38,56.06 23.9,22.86 33.66,49.78 33.66,48.89 32.38,51.05 31.62,50.55 38.23,53.59 39.24,53.59 40.89,53.59 42.04,53.59 43.18,53.59 43.31,49.91 44.2,48.77 32.26,46.89 32,48.67 29.46,52.58 29.46,53.59 30.1,53.09 30.86,53.59 31.62,54.1 32.64,54.61 33.66,54.99 34.54,55.24 35.56,55.5 36.45,55.63 37.72,55.75 27.18,53.21 26.8,52.45 26.42,51.56 25.65,50.55 27.05,54.36 26.92,55.24 37.49,54.6 23.98,58.84 23.98,59.86 23.98,60.74 23.98,61.63 23.98,62.52 17.3,56.69 17.3,57.58 17.3,58.47 17.35,53.01 17.98,54.41 17.35,52.12 19.2,50.9 18.67,49.15 16.94,47.24 12.19,47.5 13.08,47.5 14.1,47.5 14.99,47.5 16,47.5 20.7,63.17 26.67,62.53 22.23,62.15 22.48,59.74 21.21,61.13 26.29,60.88 26.04,53.77 30.73,55.04 0.64,47.42 4.57,47.16 47.54,62.99 45.34,62.99 45.72,63.63 46.61,63.63 43.85,63.65 44.7,63.5 17.91,45.97 18.14,48.56 18.87,49.71 30.1,68.58 31.37,68.58 32.51,68.58 33.66,68.58 34.92,68.58 36.07,68.58 37.21,68.58 38.61,68.58 39.75,68.58 40.89,68.58 42.16,68.58 43.43,68.58 44.58,68.58 30.1,66.17 31.37,66.17 32.64,66.17 33.91,66.17 35.05,66.17 30.1,64.77 31.37,64.77 32.51,64.77 33.53,64.77 34.67,64.77 38.35,65.28 37.72,64.14 37.97,66.68 36.45,67.06 40.01,65.79 41.66,65.91 42.93,65.91 44.07,65.91 45.34,66.04 46.74,66.04 40.39,64.26 42.42,64.52 40.51,67.18 42.93,67.31 44.96,67.31 34.29,67.31 32.26,67.31 30.48,67.31 32.89,58.8 35.69,59.18 38.99,59.18 41.53,58.29 34.67,61.47 36.45,61.47 38.35,61.47 40.13,61.47
  pour Top (no thermals): 22.61,15.49 23.5,15.49 23.88,15.11 23.88,12.45 23.75,12.32 22.61,12.32 22.48,12.45 22.48,15.37
  pour Route2 (rank 6): 1.27,71.04 47.62,71.04 48.9,65.15 48.9,-3.43 47.62,-4.7 0.64,-4.7 -1.27,-2.79 -1.27,63.88
  pour Top (isolate 0.152, rank 6): 1.27,71.04 47.62,71.04 48.9,65.15 48.9,-1.52 46.99,-3.43 0.76,-3.43 -1.27,-1.4 -1.27,63.88
  pour Bottom (rank 6): 1.27,71.04 47.62,71.04 48.9,65.15 48.9,-4.7 46.35,-7.24 1.91,-7.24 -1.27,-4.06 -1.27,63.88
  pour Route15 (rank 6): 1.27,71.04 47.62,71.04 48.9,65.15 48.9,-4.7 47.62,-5.97 0.64,-5.97 -1.27,-4.06 -1.27,63.88
GNSS_PWR
  Top 0.152: R6.2 L7.2 19.87,48.69 arc-45 ANT2.D
INT1  (via drill 0.25 pad 0.51)
  Top 0.152: U7.11 38.35,50.8 v38.23,50.67 | v37.66,48.01 37.66,48.5 R30.1 | v30.48,42.8 30.48,43.64 U1.56
  Route15 0.152: v38.23,50.67 38.23,48.58 v37.66,48.01 31.75,48.01 30.48,46.74 v30.48,42.8
INT2  (via drill 0.25 pad 0.51)
  Top 0.152: U7.9 39.1,49.8 39.62,49.28 40.26,49.28 40.47,49.07 R31.1 40.51,48.47 v40.51,47.5 | U1.58 28.62,43.26 29.08,42.8 29.59,42.8 v29.84,42.55
  Route15 0.152: v29.84,42.55 30.1,42.29 30.86,42.29 31.11,42.55 31.11,46.48 32.13,47.5 v40.51,47.5
LNA_CTL  (via drill 0.25 pad 0.51)
  Top 0.152: R10.2 31.7,45.22 31.19,44.78 29.72,44.78 29.52,44.51 U1.57 | U3.6 27.39,58.01 v27.3,58.09
  Top 0.156: R10.2 v32.38,45.97 | C32.2 27.01,58.09 v27.3,58.09
  Bottom 0.152: 28.83,50.42 28.83,56.05 28.19,56.69
  Bottom 0.156: v32.38,45.97 29.59,45.97 28.83,46.74 28.83,50.42 | 28.19,56.69 27.3,57.58 v27.3,58.09
LR_DIO9
  Top 0.156: U1.11 13.38,33.1 13,33.48 R7.2
N$1
  Top 0.156: USB1.A5 25.42,7.77 R1.2
N$2
  Top 0.156: USB1.B5 28.42,8.1 R2.2
N$3
  Top 0.152: 18.46,56.69 R3.2 | 18.49,57.56 C1.2
  Top 0.156: C1.2 18.46,56.69 | L1.1 18.49,57.56
N$4
  Top 0.152: C2.2 | 16.76,61.72 16.3,61.72 ANT6.1
  Top 0.156: L1.2 C2.2 | C2.2 17.72,60.89 16.76,61.72
N$5
  Top 0.152: U1.72 arc-90 16,43.72 | 18.41,55.64 R4.1
  Top 0.156: 16,43.72 16,44.46 arc-45 16.09,44.66 16.66,45.24 arc45 17.53,47.32 17.53,48.26 arc-45 17.98,49.34 arc45 18.5,50.61 18.5,55.41 R4.1
N$6
  Top 0.156: L2.1 28.4,63.28 C3.2 28.4,61.65 C34.1
N$7
  Top 0.152: Q1.3 33.99,16.43
  Top 0.156: Q2.1 34.16,15.62 R24.1 33.99,16.43
N$8
  Top 0.152: Q4.1 29.47,49.27 R12.1 31.19,49.53 Q3.3
N$9
  Top 0.152: R10.1 30.79,45.99 R27.2 30.79,47.67 Q3.1
N$10
  Top 0.305: JP1.1 14.9,19.73 D3.+
N$11
  Top 0.152: Q1.1 33.97,18.87
  Top 0.156: 33.97,18.87 R26.2 33.97,20.68 R23.1
N$12  (via drill 0.25 pad 0.51)
  Top 0.156: U1.65 22.35,43.73 v22.35,45.85 | C5.2 22.71,64.92 L5.1 22.71,64.95 v24.51,64.95
  Bottom 0.156: v24.51,64.95 24.51,51.06 arc-45 v22.35,45.85
N$13
  Top 0.156: U1.29 25.02,24 24.69,23.67 X1.2 24.69,22.61 24.69,22.43 24.69,21.88 C17.2
N$14  (via drill 0.25 pad 0.51)
  Top 0.152: R21.1 v28.32,22.1 | v13.97,22.1 13.97,21.08 13.34,20.45 13.34,11.18 6.86,4.7 6.86,1.93 D4.-
  Bottom 0.152: v28.32,22.1 v13.97,22.1
N$15
  Top 0.156: 20.8,66.34 C6.2 20.8,64.97 L5.2
  Top 0.635: ANT3.1 22.16,67.7 arc90 20.8,66.34
N$16
  Top 0.152: 26.98,48.8 27.27,49.25
  Top 0.156: L6.1 41.02,55.04 C7.2 arc66 27.27,49.25 | 26.98,48.8 24.55,45.07 arc33 U1.63
N$17
  Top 0.156: U1.30 25.92,23.99 26.31,23.6 X1.1 26.31,21.95 C20.2
N$18
  Top 0.156: L6.2 43.01,54.99 | 43.01,54.99 C8.2 | 43.01,54.99 45.09,54.99
  Top 0.635: ANT4.2 46.42,56.32 arc-90 45.09,54.99
N$19
  Top 0.635: C9.2 ANT3.3 | C9.2 27.61,68.63 25.65,68.63 | C9.2 27.61,67.68 25.59,67.68
N$20
  Top 0.156: C10.2 46.89,62.13 46.86,62.1
  Top 0.635: 46.48,60.07 46.51,60.05 ANT4.3 46.89,62.08 46.86,62.1 | 46.48,60.07 46.48,62.1 46.86,62.1 | 46.86,62.1 47.37,62.1 47.37,60.07 46.86,60.07 | 46.48,60.07 46.42,60.07 46.42,62.1 46.48,62.04 46.74,62.04
N$21
  Top 0.152: 20.55,55.73 ANT1.D
  Top 0.156: R4.2 20.55,55.73
N$22
  Top 0.254: D5.- 10.03,1.02 10.54,1.42 R22.1
N$23
  Top 0.156: L2.2 28.33,64.18 C4.2 arc-45 29.05,65.42 ANT5.1
N$24
  Top 0.156: R5.2 21.21,46.68 arc22 24.43,48.43 arc49 U3.3
N$25
  Top 0.156: U1.67 R6.1 | R6.1 20.57,45.97 | 20.57,45.97 | 20.57,45.97 R6.1 | R6.1 R5.1
N$26
  Top 0.305: U5.3 19.86,15.03 19.94,15.11 19.94,15.75 20.07,15.88 20.07,16
  pour Top (no thermals): 19.3,15.62 20.7,17.02 21.34,17.02 21.34,16.51 20.57,16.13 19.94,15.62 19.81,15.49 19.3,15.49
N$27  (via drill 0.25 pad 0.51)
  Top 0.254: Q4.3 28.37,46.05 C33.2 v27.61,45.62 | L7.1 18.92,47.73 v18.92,47.12
  Bottom 0.254: v27.61,45.62 25.45,45.62 24.64,44.96 19.18,44.96 18.92,45.21 v18.92,47.12
N$28
  Top 0.305: 18.89,12.74 19.05,12.57 | 19.05,12.57 19.18,12.45 | 19.18,12.45 19.18,11.43 | 19.05,12.57 19.05,11.43 | 19.18,12.45 19.18,13.08 19.05,13.21 U5.16 18.89,12.74 | 18.89,12.74 18.89,11.52 18.54,11.18 | U5.14 17.89,12.09 C25.1 17.86,11.13 17.78,11.05
  Top 0.762: J2.+ 14.37,10.3 15.11,11.05 17.78,11.05 18.8,11.05 19.18,11.43
N$29
  pour Top (no thermals): 27.3,13.72 29.84,13.72 30.1,13.46 30.1,12.7 28.57,12.7 28.57,13.08 27.76,13.51 27.38,13.51 27.3,13.59
N$30
  Top 0.152: R17.1 16.82,18.16 16.21,18.16 D3.-
N$31
  Top 0.152: U5.9 16.66,15.9 16.89,16.13 R17.2
N$32  (via drill 0.25 pad 0.51)
  Top 0.254: R29.2 C35.1 | C35.1 R28.1 | v29.57,18.64 29.99,18.64 C35.1
  Top 0.305: U6.4 27.57,14.62 27.81,14.86 v28.07,14.86
  Bottom 0.254: v28.07,14.86 28.19,14.99 29.57,16.23 v29.57,18.64
N$33
  Top 0.152: U5.7 17.89,17.19 R18.1 R16.2
N$34
  Top 0.152: U5.11 16.09,14.53 R20.1
N$35
  Top 0.156: L8.1 28.38,58.02 U3.5
N$36
  Top 0.152: U5.12 16.48,14.03 R19.1
N$37
  Top 0.152: U5.5 18.89,16.67 R15.1
N$39
  cutout Top: 44.96,54.61 44.96,62.61 48.01,62.61 48.01,54.61
  cutout Route2: 44.96,54.61 44.96,62.61 48.01,62.61 48.01,54.61
  cutout Bottom: 44.96,54.61 44.96,62.61 48.01,62.61 48.01,54.61
  cutout Route15: 44.96,54.61 44.96,62.61 48.01,62.61 48.01,54.61
N$40
  cutout Top: 21.08,54.48 21.08,56.9 23.11,56.9 23.11,54.48
  cutout Route2: 21.08,54.48 21.08,56.9 23.11,56.9 23.11,54.48
  cutout Bottom: 21.08,54.48 21.08,56.9 23.11,56.9 23.11,54.48
  cutout Route15: 21.08,54.48 21.08,56.9 23.11,56.9 23.11,54.48
N$41
  cutout Top: 20.32,69.26 28.32,69.26 28.32,66.22 20.32,66.22
  cutout Route2: 20.32,69.26 28.32,69.26 28.32,66.22 20.32,66.22
  cutout Bottom: 20.32,69.26 28.32,69.26 28.32,66.22 20.32,66.22
  cutout Route15: 20.32,69.26 28.32,69.26 28.32,66.22 20.32,66.22
N$42
  Top 0.152: L8.2 28.37,59.86
  Top 0.156: 28.37,59.86 C34.2
N$43
  cutout Top: -1.4,69.77 17.91,69.77 17.91,61.01 -1.27,61.01
  cutout Route2: -1.4,69.77 17.91,69.77 17.91,61.01 -1.27,61.01
  cutout Route15: -1.4,69.77 17.91,69.77 17.91,61.01 -1.27,61.01
  cutout Bottom: -1.4,69.77 17.91,69.77 17.91,61.01 -1.27,61.01
N$44
  cutout Top: 16.89,61.01 16.89,48.01 -0.51,48.01 -0.51,61.01
  cutout Route2: 16.89,61.01 16.89,48.01 -0.51,48.01 -0.51,61.01
  cutout Route15: 16.89,61.01 16.89,48.01 -0.51,48.01 -0.51,61.01
  cutout Bottom: 16.89,61.01 16.89,48.01 -0.51,48.01 -0.51,61.01
N$45
  cutout Top: 21.08,49.15 21.08,51.56 23.11,51.56 23.11,49.15
  cutout Route2: 21.08,49.15 21.08,51.56 23.11,51.56 23.11,49.15
  cutout Bottom: 21.08,49.15 21.08,51.56 23.11,51.56 23.11,49.15
  cutout Route15: 21.08,49.15 21.08,51.56 23.11,51.56 23.11,49.15
N$47
  cutout Top: 17.91,61.01 17.78,61.01 16.89,61.01 16.89,60.07 17.91,60.07 18.45,60.75 18.45,69.77 17.91,69.77
  cutout Bottom: 17.91,61.01 17.78,61.01 16.89,61.01 16.89,60.07 17.91,60.07 18.45,60.75 18.45,69.77 17.91,69.77
  cutout Route15: 17.91,61.01 17.78,61.01 16.89,61.01 16.89,60.07 17.91,60.07 18.45,60.75 18.45,69.77 17.91,69.77
  cutout Route2: 17.91,61.01 17.78,61.01 16.89,61.01 16.89,60.07 17.91,60.07 18.45,60.75 18.45,69.77 17.91,69.77
NRF_DN
  Top 0.142: U1.40 33.31,29.5 33.6,29.79 34.57,29.79 34.8,29.57 34.8,24.33 34.59,24.13 34.29,24.13 34.16,24 34.16,23.7 33.96,23.49 33.66,23.49 33.4,23.24 33.4,22.99 33.15,22.73 32.89,22.73 32.64,22.48 32.64,22.17 32,21.54 32,13.59 30.35,11.94 26.8,11.94 26.52,11.66 26.52,11.23 R11.2
NRF_DP
  Top 0.142: 33.25,30.4 33.55,30.1 34.67,30.1 35.1,29.67 35.1,24.18 32.31,21.39 32.31,13.45 30.49,11.63 26.92,11.63 26.82,11.53 26.82,11.23 R13.2
  Top 0.156: 33.25,30.4 U1.41
P0.02
  Top 0.156: U1.12 13.39,32.2 13.08,32.51 12.32,32.51 R7.1
P0.04/SCL  (via drill 0.25 pad 0.51)
  Top 0.152: U4.2 33.17,46.21 v32.89,46.48 32.89,49.91 33.66,50.67 35.43,50.67 35.81,50.3 U7.4
  Top 0.156: 37.92,16.64 J8.1 38,19.15 v37.72,19.43 R14.1 | 26.8,25.18 U1.31 26.82,24.36 27.43,23.75 v27.43,22.61 v27.43,20.32
  Route15 0.152: v32.89,46.48 32.89,35.69 30.86,33.66 30.86,28.07 30.1,27.3 30.1,23.24 29.46,22.61 v27.43,22.61
  Bottom 0.156: v27.43,20.32 35.56,20.32 36.45,19.43 v37.72,19.43
P0.05/SDA  (via drill 0.25 pad 0.51)
  Top 0.152: U7.6 37.09,48.39 36.7,48.01 34.29,48.01 33.92,47.64 U4.1 33.42,47.01 v33.4,46.99
  Top 0.156: 14.41,27.69 U1.17 13.48,27.7 13.34,27.56 v13.34,21.59 | 37.89,14.61 J8.2 39.73,14.72 40.01,14.99 40.01,19.69 39.37,20.32 v37.72,20.32 R25.1
  Route15 0.152: v33.4,46.99 33.4,35.43 31.37,33.4 31.37,27.81 30.61,27.05 30.61,22.35 29.84,21.59 v26.92,21.59
  Bottom 0.156: v13.34,21.59 v26.92,21.59 27.56,20.95 35.81,20.95 36.45,20.32 v37.72,20.32
P0.06/LED_BLUE
  Top 0.152: 27.69,25.24 U1.32 27.72,24.3 R21.2
P0.13/D0_1  (via drill 0.25 pad 0.51)
  Top 0.156: U1.39 32.95,28.58 v34.04,28.58 | v7.75,28.58 7.75,38.1 8.3,38.66 J4.1
  Bottom 0.156: v34.04,28.58 v7.75,28.58
P0.14/D0_2  (via drill 0.25 pad 0.51)
  Top 0.156: U1.38 32.94,27.69 v34.04,27.69 | v7.11,27.69 7.11,39.88 7.89,40.66 J4.2
  Bottom 0.156: v34.04,27.69 v7.11,27.69
P0.15/D1_1  (via drill 0.25 pad 0.51)
  Top 0.156: U1.42 32.06,31.3 31.5,30.73 v31.5,27.05 | J7.1 11.18,24.36 v11.18,25.65
  Bottom 0.156: v31.5,27.05 11.56,27.05 11.18,26.67 v11.18,25.65
P0.16/D1_2  (via drill 0.25 pad 0.51)
  Top 0.156: U1.26 22.35,25.23 v22.35,26.29 | J7.2 10.05,26.29 v11.81,26.29
  Bottom 0.156: v22.35,26.29 v11.81,26.29
P0.24/RXD  (via drill 0.25 pad 0.51)
  Top 0.156: U1.47 32.93,35.81 v33.91,35.81 | J3.1 37.95,30.73 37.97,30.76 v37.97,35.81
  Bottom 0.156: v37.97,35.81 v33.91,35.81
P0.25/TXD  (via drill 0.25 pad 0.51)
  Top 0.152: 39.73,28.69 40.01,28.96 40.01,37.34 40.64,37.97 v40.64,40.26
  Top 0.156: U1.52 32.97,40.26 v34.04,40.26 | J3.2 37.89,28.58 | J3.2 38.85,28.69 | J3.2 39.73,28.69
  Bottom 0.156: v34.04,40.26 v40.64,40.26
P0.28/AIN4  (via drill 0.25 pad 0.51)
  Top 0.156: U1.14 14.37,30.35 v13.34,30.35 | J6.1 36.02,44.66 35.56,44.2 v34.54,44.2
  Bottom 0.152: 12.83,35.18 12.83,41.27 15.75,44.2 v34.54,44.2
  Bottom 0.156: v13.34,30.35 12.83,30.86 12.83,35.18
P0.29/AIN5  (via drill 0.25 pad 0.51)
  Top 0.156: U1.9 14.4,34.92 v13.46,34.92 | v34.04,43.69 36.07,43.69 37.1,42.66 J6.2
  Bottom 0.152: v13.46,34.92 13.46,41.15 16,43.69 v34.04,43.69
P0.30/D2_1
  Top 0.156: U1.15 13.5,29.5 12.83,28.83 12.83,11.3 12.24,10.72 J5.1
P0.31/D2_2
  Top 0.156: U1.10 11.9,34 11.43,33.53 11.43,32.38 12.32,31.5 12.32,12.95 12.08,12.72 J5.2
P1.01/EN_3V3
  Top 0.152: U1.54 34.99,42.1 35.56,41.53 35.56,39.5 36.2,38.86 | 35.81,25.53 35.81,30.73 37.34,32.26 37.34,36.7 36.45,37.59
  Top 0.156: U1.54 32.98,42.16 | 35.81,25.53 35.81,23.62 33.07,20.87 R23.2 | 36.45,37.59 36.32,37.72 36.32,38.73 36.2,38.86
P1.02/USER
  Top 0.152: U1.55 31.6,44.38 32.74,45.47 39.88,45.47 41.15,44.2 41.15,37.59 40.51,36.96 40.51,8.64 | 34.37,5.54 34.16,5.33 34.16,5.21 33.86,4.9 K1.3 K1.4
  Top 0.156: 34.37,5.54 C28.2 | C28.2 R9.1 35.35,6.14 | U1.55 31.37,43.75 | 40.51,8.64 39.88,8 35.31,8 34.37,7.07 C28.2
QSPI_CS
  Top 0.156: U1.45 33.69,34 34.5,33.19 U2.1
QSPI_DATA0
  Top 0.152: 34.04,32.13 35.31,32.13 35.56,31.88 36.32,31.88 36.96,32.51 36.96,35.69 36.75,35.89 U2.5
  Top 0.156: U1.43 32.99,32.13 34.04,32.13 | U2.5
QSPI_DATA1
  Top 0.156: U2.2 35.44,33.91 35.31,34.04 34.54,34.04 33.68,34.9 U1.46
QSPI_DATA2  (via drill 0.25 pad 0.51)
  Top 0.156: U1.53 32.99,41.27 v33.91,41.27 | U2.3 v35.94,32.38
  Bottom 0.152: v33.91,41.27 33.53,41.27 33.15,40.89 33.15,32.89 33.66,32.38 v35.94,32.38
QSPI_DATA3
  Top 0.152: U2.7 35.44,38.1 35.31,38.23 35.18,38.23
  Top 0.156: U1.49 32.93,37.59 33.78,37.59 34.42,38.23 35.18,38.23 | U2.7
QSPI_SCK  (via drill 0.25 pad 0.51)
  Top 0.152: U2.6 35.94,38.48 34.8,39.62 v34.8,41.27
  Top 0.156: U1.61 25.91,43.72 v25.91,44.7
  Bottom 0.156: v25.91,44.7 35.43,44.7 35.69,44.45 35.69,43.94 34.8,43.05 v34.8,41.27
RST  (via drill 0.25 pad 0.51)
  Top 0.152: v42.67,39.75 v42.67,48.39 | R8.1 39.45,5.54 38.94,5.03 K2.3
  Top 0.156: U1.36 31.37,25.16 v31.37,24.13 | K2.4 K2.3 | R8.1 C29.2 40.43,7.16 42.22,9.45 42.22,26.49 v43.59,27.86
  Bottom 0.152: 40.31,27.74 CN1.10 43.48,27.74 | 43.48,27.74 43.94,28.19 43.94,33.53 42.67,34.8 v42.67,39.75 | 43.48,27.74 43.48,27.76 v43.59,27.86 | J1.3 37.59,48.89 38.1,48.39 v42.67,48.39
  Bottom 0.156: 40.31,27.74 39.24,26.67 39.24,24.77 38.61,24.13 v31.37,24.13
SWDCLK  (via drill 0.25 pad 0.51)
  Top 0.152: v41.66,39.37 v41.66,52.32
  Top 0.156: U1.51 32.95,39.37 v34.04,39.37
  Bottom 0.152: CN1.4 42.98,31.55 43.56,32.13 43.56,33.27 42.29,34.54 42.29,39.12 42.04,39.37 v41.66,39.37 v34.04,39.37 | J1.4 38.64,52.32 v41.66,52.32
SWDIO  (via drill 0.25 pad 0.51)
  Top 0.152: v41.78,38.48 42.16,38.86 v42.16,51.82
  Top 0.156: U1.50 32.94,38.48 v33.91,38.48
  Bottom 0.152: CN1.2 41.78,33.02 v41.78,38.48 41.02,38.48 | J1.2 38.86,51.3 39.37,51.82 v42.16,51.82
  Bottom 0.156: v33.91,38.48 41.02,38.48
SWO/TRACEDATA0  (via drill 0.25 pad 0.51)
  Top 0.152: v41.15,36.7 v43.18,36.7 43.18,48.64 42.67,49.15 v42.67,52.83
  Top 0.156: U1.48 | U1.48 v33.91,36.7
  Bottom 0.152: CN1.14 43.48,25.2 44.32,26.03 44.32,33.91 43.18,35.05 v43.18,36.7 | J1.6 36.32,51.43 37.72,52.83 v42.67,52.83
  Bottom 0.156: v33.91,36.7 v41.15,36.7
TRACECLK  (via drill 0.25 pad 0.51)
  Top 0.156: U1.19 16,25.18 v16,24
  Bottom 0.152: 40.31,26.47 CN1.12
  Bottom 0.156: v16,24 30.35,24 30.86,23.49 38.99,23.49 40.01,24.51 40.01,26.16 40.31,26.47
TRACEDATA1  (via drill 0.25 pad 0.51)
  Top 0.152: 30.48,25.15 30.48,23.75 v31.37,22.86
  Top 0.156: U1.35 30.48,25.15
  Bottom 0.156: v31.37,22.86 39.24,22.86 40.31,23.93 CN1.16
TRACEDATA2  (via drill 0.25 pad 0.51)
  Top 0.156: v21.46,23.49 21.46,25.16 U1.25
  Bottom 0.156: v21.46,23.49 29.46,23.49 30.73,22.23 39.62,22.23 40.06,22.66 CN1.18
TRACEDATA3  (via drill 0.25 pad 0.51)
  Top 0.156: U1.34 29.59,25.13 v29.59,22.1
  Bottom 0.152: 39.75,21.59 30.1,21.59 v29.59,22.1
  Bottom 0.156: 39.75,21.59 39.95,21.39 CN1.20
USB_DN
  Top 0.142: R11.1 26.52,9.6 26.52,8.36 26.3,8.13 25.91,8.13 | D2.1 25.91,7.37 | 25.91,7.37 25.91,6.23 USB1.B7 | USB1.A7 26.92,7.24 26.8,7.37 25.91,7.37
  Top 0.156: 25.91,8.13 D2.1 25.92,8.27
USB_DP
  Top 0.142: R13.1 26.82,9.6 26.82,8.36 27.05,8.13 27.43,8.13 | 27.43,8.25 27.43,8.13 | 27.43,8.13 D1.1 27.43,6.23 USB1.B6 27.42,5.32 27.3,5.21 26.54,5.21 26.42,5.33 USB1.A6
  Top 0.156: D1.1
VBUS  (via drill 0.25 pad 0.51)
  Top 0.508: v30.23,7.49 v29.72,7.49 29.46,7.49 29.07,7.1 USB1.B4_A9 | 24.27,7.06 24.27,7.48 | 24.27,7.48 24.26,7.49 v24.13,7.49 | v24.13,7.49 23.83,7.49 | 23.83,7.49 v23.62,7.49 F1.1 | 24.27,7.06 23.83,7.49 | 24.27,7.48 24.27,9.38 F1.1 | F1.1 23.88,9.78 23.88,7.75 v24.13,7.49 | 24.27,7.06 USB1.A4_B9
  Bottom 0.508: v30.23,7.49 v24.13,7.49 v23.62,7.49
VDD_LR
  Top 0.508: U1.22 18.72,24.44 18.41,24.13 18.41,24 | 18.41,24 C15.2 C14.2 18.33,22.27 C16.2 18.03,20.36 FB2.1 18.19,20.52 | U1.21 17.82,24.59 18.41,24
VDD_NRF
  Top 0.305: C11.2 23.11,23.75
  Top 0.508: C11.2 23.22,23.86 U1.27 | U1.28 24.12,24.68 C11.2 | C11.2 C12.2 23.2,22.27 C13.2 23.5,20.36 FB1.1
VSYS
  Top 0.152: U5.1 19.68,14.01 19.68,13.84
  Top 0.254: U5.15 18.39,13.69 18.73,14.03 U5.1
  Top 0.305: U6.7 24.54,13.62 | C21.2 25.3,17.04 25.27,17.02 25.27,18.16 24,19.43 17.14,19.43 JP1.2
  Top 0.381: 24.54,13.62 24.51,13.59 | U6.8 24.55,13.12 24.51,13.08 | 20.64,12.93 20.22,12.93 19.68,13.46 19.68,13.84 19.81,13.84 19.81,13.46 20.07,13.21 20.91,13.21 | 20.64,12.93 C24.1 | 20.64,12.93 20.91,13.21 | 20.91,13.21 20.95,13.21
  Top 0.762: C24.1 21.31,12.06 21.31,11.84 21.59,11.56 24,11.56 24.51,12.06 24.51,13.08 24.51,13.59 24.51,14.48 | 24.51,14.48 24.51,15.27 | 24.51,14.48 25.02,14.99
  pour Top (no thermals): 22.48,17.78 25.53,17.78 25.78,17.53 25.78,14.73 25.58,14.53 24.97,14.53 22.48,17.02
VUSB  (via drill 0.25 pad 0.51)
  Top 0.254: R16.1 18.67,18.11 v18.67,18.8
  Top 0.305: U1.37 v34.04,26.8 | v15.11,22.73 15.11,21.46 13.97,20.07 13.97,17.91 14.83,17.05 C23.1
  Top 0.381: U5.2 20.5,14.53 v20.5,14.61
  Bottom 0.254: v18.67,18.8 18.67,17.02
  Bottom 0.305: v34.04,26.8 34.04,25.78 33.66,25.4 23.88,25.4 23.75,25.4 16.26,25.4 15.75,24.89 15.43,24.57 15.11,24.26 v15.11,22.73
  other vias: 16.13,17.27 16.13,16.64 20.5,15.11 20.07,10.29 20.07,9.65
  pour Top (no thermals): 14.61,17.53 16.38,17.53 16.38,16.38 14.48,16.38 14.48,17.53
  pour Top (no thermals): 21.46,15.49 20.32,15.37 20.32,14.35 21.72,14.22 21.72,15.49
  pour Bottom: 15.75,17.65 19.05,17.65 20.95,15.75 20.95,14.35 20.83,14.22 20.19,14.22 20.07,14.35 20.07,15.37 19.56,15.88 19.18,16.26 16.26,16.26 15.88,16.26 15.75,16.38 15.62,16.51 15.62,16.89 15.62,17.53
  pour Top (no thermals): 21.84,10.67 19.68,10.67 19.68,9.14 21.84,9.14
  pour Bottom (no thermals): 20.07,14.35 20.07,13.46 20.32,13.21 20.7,12.83 20.7,12.06 20.7,11.56 19.81,10.67 19.68,10.54 19.68,9.53 19.94,9.27 20.19,9.27 20.45,9.53 20.45,10.03 20.83,10.41 21.34,10.92 21.34,12.45 21.34,13.59 21.08,13.84 20.95,13.97 20.95,14.86 20.95,15.37 20.83,15.49 20.32,15.49 20.19,15.37 20.07,15.24

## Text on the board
tPlace: Wi-Fi | GNSS | LoRa | BLE | Z | X | LoRa | Y | GNSS | TH | GND | A4 | 28 | A5 | 29 | 3V3 | Digital0 | 14 | 3V3 | Analog | 13 | GND | GND | RX | 24 | TX | 25 | 3V3 | 16 | 3V3 | UART | Digital1 | 15 | GND | CHARGE | GND | SCL | 4 | 3V3 | SDA | 5 | I2C | 31 | 3V3 | Digital2 | - | 30 | + | BAT | GND | LED | GROVE | BUTTON | RESET
bPlace: SWD | SWD+Trace | Wio Tracker 1110 | v1.0 8/22/2023 | LiPo | 3.7V | + | -
tNames: LAYER STACK-UP - ALL DIMENSIONS IN MIL | L1-L2: 3.91mil | 50ohm SINGLE ENDED / IMPEDANCE CONTROL +/-10% | 90ohm SINGLE ENDED / IMPEDANCE CONTROL +/-10% | TRACE WIDTH (mil) | TRACE WIDTH / SPACE (mil) | LAYER# | COPPER WEIGHT / (OZ) | LAYER 1 - GTL | HALF+PLATING=1OZ | 6.16 | 5.59/6 | LAYER 2 - GND | HALF=0.5OZ | LAYER 3 - POWER | HALF=0.5OZ | LAYER 4 - GBL | HALF+PLATING=1OZ | 6.16 | 5.59/6
tTest: ANT5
